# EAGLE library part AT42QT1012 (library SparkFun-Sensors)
Atmel AT42QT1010 1-Channel Capacitive Touch Sensor The AT42QT1010 is a dedicated, single-button capacitive sense chip. The chip handles monitoring a conductive area for touch. As long as a touch (e.g. from a finger) is detected, the AT42QT1010 keeps the output line high. Otherwise, the line is kept low. Datasheet SparkFun Products SparkFun Capacitive Touch Breakout - AT42QT1010 (SEN-12041)
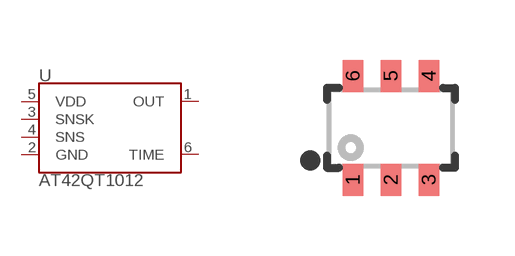
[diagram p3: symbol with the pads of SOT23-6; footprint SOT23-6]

Designator prefix U

## AT42QT1012-TSHR (PROD_ID: IC-11778)  [SOT23-6]
1  OUT
2  GND
3  SNSK
4  SNS
5  VDD
6  TIME

## Footprint SOT23-6 (pad centres in mm)
6-Pin SOT23-6 Datasheet Specifications: Pin Count: 6 Area: 2.6 x 2.9 x 1.45 mm Pitch: 0.95 mm Devices Using: AT42QT1012
smd 0.51 x 0.8: 1 -0.95,-1.3; 2 0,-1.3; 3 0.95,-1.3; 4 0.95,1.3; 5 0,1.3; 6 -0.95,1.3

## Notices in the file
Licensing: Creative Commons ShareAlike 4.0 International - https://creativecommons.org/licenses/by-sa/4.0
